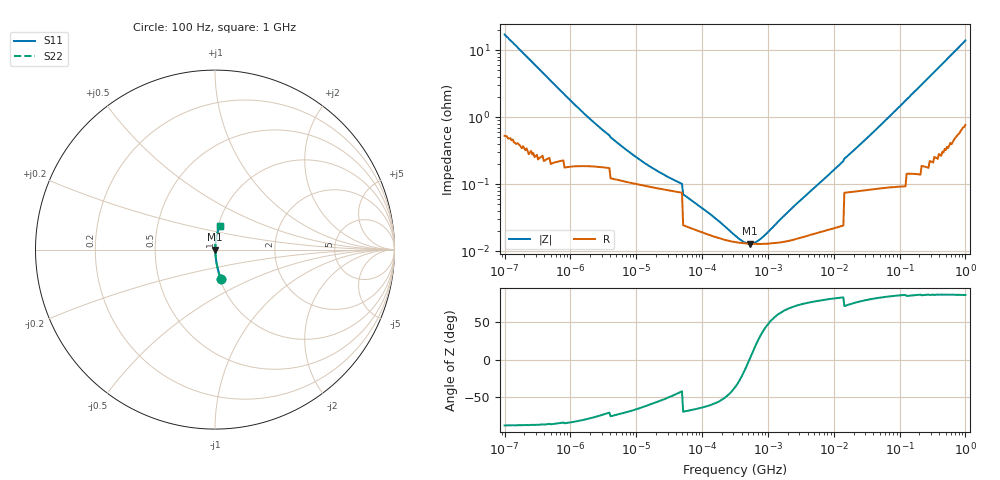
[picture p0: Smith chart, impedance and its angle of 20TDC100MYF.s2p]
!  *** S-Parameter ***
!  Copyright (C) Panasonic Industry Corporation
!  Conductive Polymer Tantalum Solid Capacitor (POSCAP)
!  Parts No. 20TDC100MYF
!  Connection Mode : Series
!  1  o---||---o  2
!  GND o--------o GND
!  Conditions : Temperature = 20   DC Bias = 0 V
! Frequency Range : 100 Hz  -  1 GHz  [ 401 Steps ]
# Hz S RI R 50
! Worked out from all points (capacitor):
!   401 points, 100 Hz to 1 GHz, reference 50 ohm
!   read as one part in series: C = 92.8 uF near 108 Hz
!   lowest |Z| = 13 mohm at 534 kHz (marker M1)
!   series resonance near 523.3 kHz, so ESL is about 1 nH
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100  0.0331 -0.164  0.967 0.164  0.967 0.164  0.0331 -0.164
169  0.0139 -0.1  0.986 0.1  0.986 0.1  0.0139 -0.1
309  0.00574 -0.0558  0.994 0.0558  0.994 0.0558  0.00574 -0.0558
1490  0.00201 -0.012  0.998 0.012  0.998 0.012  0.00201 -0.012
2830  0.00169 -0.00664  0.998 0.00664  0.998 0.00664  0.00169 -0.00664
5620  0.00131 -0.0037  0.999 0.0037  0.999 0.0037  0.00131 -0.0037
10700  0.000995 -0.00219  0.999 0.00219  0.999 0.00219  0.000995 -0.00219
22100  0.000723 -0.00126  0.999 0.00126  0.999 0.00126  0.000723 -0.00126
49500  0.0005 -0.000685  0.999 0.000685  0.999 0.000685  0.0005 -0.000685
102000  0.000381 -0.00039  1 0.00039  1 0.00039  0.000381 -0.00039
211000  0.0003 -0.000194  1 0.000194  1 0.000194  0.0003 -0.000194
329000  0.000273 -9.53e-05  1 9.53e-05  1 9.53e-05  0.000273 -9.53e-05
534000  0.00026 4.21e-06  1 -4.21e-06  1 -4.21e-06  0.00026 4.21e-06
799000  0.000258 8.97e-05  1 -8.97e-05  1 -8.97e-05  0.000258 8.97e-05
1200000  0.000264 0.000189  1 -0.000189  1 -0.000189  0.000264 0.000189
1940000  0.000283 0.000344  1 -0.000344  1 -0.000344  0.000283 0.000344
4700000  0.00036 0.000812  1 -0.000812  1 -0.000812  0.00036 0.000812
1.4e7  0.000495 0.0022  1 -0.0022  1 -0.0022  0.000495 0.0022
7e7  0.000994 0.0101  0.999 -0.0101  0.999 -0.0101  0.000994 0.0101
3.24e8  0.00427 0.045  0.996 -0.045  0.996 -0.045  0.00427 0.045
5.69e8  0.00985 0.0779  0.99 -0.0779  0.99 -0.0779  0.00985 0.0779
1e9  0.026 0.134  0.974 -0.134  0.974 -0.134  0.026 0.134
